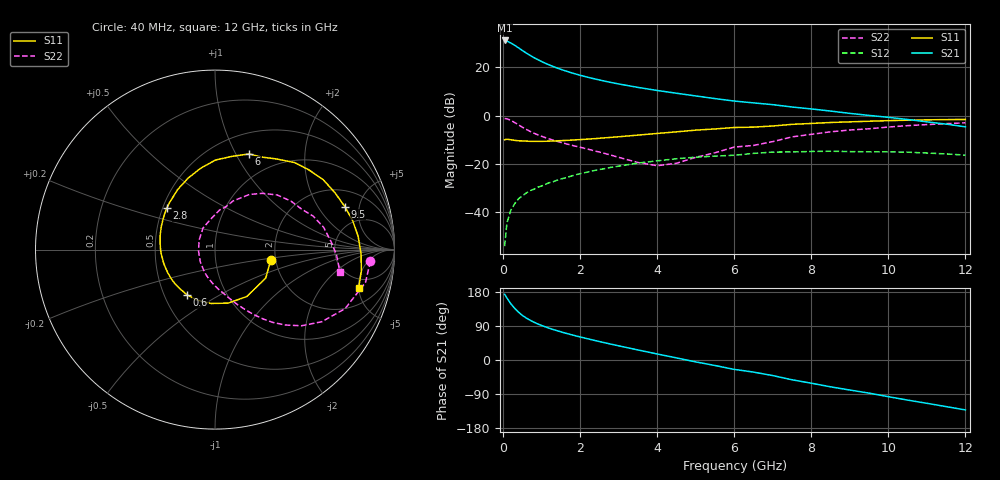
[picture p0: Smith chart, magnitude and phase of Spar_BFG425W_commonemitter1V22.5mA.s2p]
! Filename: 122bfg425.001
! BFG425W Field C1
! V1=8.780E-001V,V2=1.000E+000V, I1=3.480E-004A, I2=2.251E-002A
# GHz  S  MA  R 50
!  S11  S21  S12  S22
!Freq(GHz)  Mag  Ang  Mag  Ang  Mag  Ang  Mag  Ang
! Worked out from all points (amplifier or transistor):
!   44 points, 40 MHz to 12 GHz, reference 50 ohm
!   highest |S21| = 31.0 dB at 40 MHz (marker M1)
!   |S21| within 3 dB of that: start of sweep to 395.9 MHz
!   unconditionally stable (mu >= 1): start of sweep to 62.53 MHz; 1.072 GHz to end of sweep
!   at 700 MHz: K = 0.83, MSG = 28.0 dB, |S12| = -31.1 dB
!   at 2.4 GHz: K = 1.19, MAG = 16.2 dB, |S12| = -22.6 dB
!   at 12 GHz: K = 1.37, MAG = 2.2 dB, |S12| = -16.4 dB
!   S11 on the Smith chart (normalised r, x): 40 MHz: 1.88, -0.24; 600 MHz: 0.65, -0.36; 2.8 GHz: 0.53, +0.28; 6 GHz: 0.72, +1.13; 9.5 GHz: 3.13, +3.58; 12 GHz: 3.61, -4.99
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0.04  0.316 -10.4  35.55 173.3  0.002 71.1  0.868 -4.3
0.1  0.324 -29.0  34.53 163.7  0.006 80.4  0.858 -12.4
0.2  0.316 -55.7  31.47 148.5  0.011 73.1  0.796 -24.4
0.3  0.307 -76.1  28.36 136.5  0.015 68.2  0.718 -34.0
0.4  0.301 -94.1  25.04 126.4  0.019 64.2  0.642 -41.4
0.5  0.299 -109.7  22.09 117.8  0.022 62.0  0.574 -47.1
0.6  0.296 -121.7  19.59 110.9  0.025 60.3  0.518 -51.6
0.8  0.293 -140.4  15.75 99.8  0.03 58.4  0.432 -58.3
0.9  0.293 -147.8  14.29 95.2  0.033 57.6  0.4 -61.0
1.1  0.294 -160.2  11.99 87.3  0.038 56.1  0.349 -65.7
1.3  0.297 -170.3  10.29 80.4  0.043 54.7  0.31 -70.1
1.6  0.305 176.8  8.452 71.5  0.051 52.1  0.265 -76.2
2.2  0.326 156.5  6.173 55.9  0.068 45.5  0.202 -90.1
2.8  0.354 139.4  4.825 41.9  0.085 37.7  0.152 -108.0
3.5  0.394 121.9  3.815 26.5  0.104 27.5  0.107 -139.8
4.5  0.46 100.1  2.886 5.6  0.128 11.8  0.103 149.3
6  0.566 70.3  1.991 -24.8  0.151 -13.1  0.223 83.3
6.5  0.576 63.6  1.825 -31.9  0.165 -17.3  0.241 76.9
8.5  0.718 32.8  1.237 -70.8  0.183 -53.4  0.461 41.3
9.5  0.762 18.3  1.006 -87.4  0.178 -69.2  0.532 25.2
10.5  0.801 5.2  0.829 -105.8  0.175 -86.7  0.618 11.6
12  0.829 -15.1  0.584 -131.7  0.152 -114.4  0.708 -10.3
